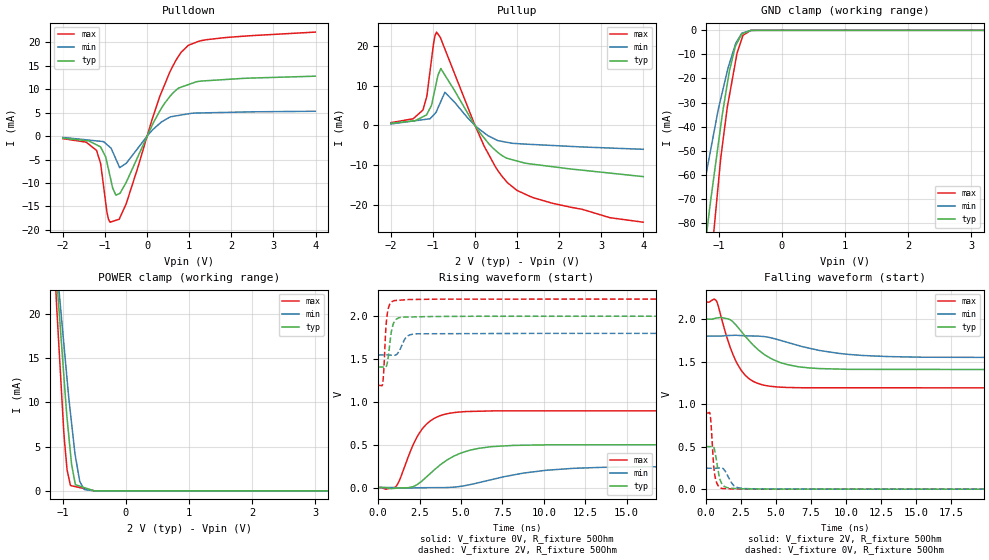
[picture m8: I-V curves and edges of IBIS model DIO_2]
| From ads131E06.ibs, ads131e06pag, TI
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|   DIO 2.0V Model
[Model]   DIO_2
Model_type   I/O
|for ADS1299 products
|Signals   SCLK, DAISY_IN
Vinl = 0.4
Vinh = 1.6
Vmeas = 1
Vref = 1
Cref = 2pF
Rref = 50
|   typ   min   max
|   (nom PVT)   (Fast PVT)   (slow PVT)
|C_comp from LC tank measurement(L=1nH)
|   (HIGH Z)
|C_comp   2.655E-12   2.033E-12   3.282E-12
|   (ON state)
C_comp   2.643E-12   2.033E-12   3.282E-12
|   (OFF state)
|C_comp   2.755E-12   2.168E-12   3.374E-12
| Where   nom PVT is  Nominal Process, 2V, 27C
|   Fast PVT is Strong Process, 2.2V, -40C
|   Slow PVT is Weak Process, 1.8V, 85C
[Voltage Range]   2   1.8   2.2
[Temperature Range]   27   85   -40
[Pullup Reference]   2   1.8   2.2
[Pulldown Reference]   0   0   0
[Power Clamp Reference]   2   1.8   2.2
[GND Clamp Reference]   0   0   0
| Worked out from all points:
|   slope of the pulldown table from 0 to 0.3 V, typ, clamps not added: 56.3 ohm
|   slope of the pullup table from 0 to 0.3 V, typ, clamps not added: 70.4 ohm
|   GND clamp passes 1 mA (typ) near -0.58 V on its own axis
|   POWER clamp passes 1 mA (typ) near -0.81 V on its own axis
|   falling waveform, V_fixture 2V, R_fixture 50Ohm: 20-80 % time 2.39ns typ, 4.11ns min, 1.41ns max; typ from 2 V to 1.41 V
|   rising waveform, V_fixture 0V, R_fixture 50Ohm: 20-80 % time 2.19ns typ, 4.04ns min, 1.33ns max; typ from 0 V to 0.501 V
|   rising waveform, V_fixture 2V, R_fixture 50Ohm: 20-80 % time 260ps typ, 390ps min, 186ps max; typ from 1.41 V to 2 V
|   falling waveform, V_fixture 0V, R_fixture 50Ohm: 20-80 % time 347ps typ, 530ps min, 235ps max; typ from 0.501 V to 0 V
[Pulldown]
|   Voltage   I(typ)   I(min)   I(max)
-2V       -446.8uA   -277.7uA   -546.8uA
-1.45V    -956.7uA   -786.1uA   -1.281mA
-1.202V   -1.858mA   -1.015mA   -3.045mA
-1.101V   -2.393mA   -1.109mA   -6.024mA
-920.3mV  -6.956mA   -2.063mA   -17.66mA
-817.4mV  -11.1mA    -3.341mA   -18.19mA
-664mV    -12.29mA   -6.482mA   -17.75mA
-496.8mV  -9.874mA   -5.806mA   -14.44mA
301.3mV   5.35mA     2.714mA    8.483mA
684.3mV   9.787mA    4.318mA    16.19mA
979.1mV   10.99mA    4.761mA    19.38mA
3.994V    12.79mA    5.303mA    22.2mA
[GND Clamp]
|   Voltage   I(typ)   I(min)   I(max)
-2V       -269mA     -184.2mA   -378.3mA
-1.355V   -119.3mA   -81.26mA   -169.4mA
-1.284V   -104.1mA   -71.39mA   -146.5mA
-1.131V   -71.25mA   -50.04mA   -99.31mA
-1.099V   -65.05mA   -45.58mA   -89.46mA
-1.009V   -47.58mA   -33.04mA   -64.31mA
-946.2mV  -35.5mA    -26.01mA   -48.62mA
-832mV    -17.03mA   -13.86mA   -27.24mA
-712mV    -5.404mA   -4.544mA   -9.78mA
-635mV    -1.555mA   -1.176mA   -3.554mA
-449.5mV  -18.29uA   -16.69uA   -19.05uA
3.994V    0A         0A         0A
[Pullup]
|   Voltage   I(typ)   I(min)   I(max)
-2V       546.5uA    370.9uA    725.3uA
-1.238V   2.207mA    1.461mA    3.888mA
-1.146V   2.755mA    1.593mA    7.345mA
-1.034V   5.103mA    2.08mA     16.64mA
-982.9mV  7.593mA    2.654mA    20.83mA
-913.5mV  11.03mA    3.622mA    23.6mA
-812.5mV  14.38mA    6.062mA    21.93mA
-716.1mV  12.74mA    8.388mA    19.32mA
210.3mV   -3.086mA   -1.805mA   -5.071mA
768.5mV   -8.32mA    -4.277mA   -14.44mA
1.417V    -9.85mA    -4.829mA   -18.36mA
3.994V    -12.92mA   -6.02mA    -24.44mA
[POWER Clamp]
|   Voltage   I(typ)   I(min)   I(max)
-2V       129.9mA    109.1mA    159.1mA
-1.265V   42.77mA    39.99mA    44.99mA
-1.099V   24.37mA    25.59mA    20.8mA
-1.077V   21.95mA    23.81mA    18.06mA
-978.4mV  12.37mA    16.1mA     5.936mA
-933.4mV  8.162mA    12.58mA    2.352mA
-879.9mV  4.267mA    8.781mA    608.5uA
-862.6mV  3.01mA     7.665mA    581.1uA
-802.3mV  700.9uA    3.939mA    485.3uA
-735.2mV  546.5uA    1.154mA    378.6uA
-660.5mV  374.8uA    150.3uA    260uA
3.994V    0A         0A         0A
[Ramp]
R_load = 50
|   typ   min   max
dV/dt_r   0.300352/2.17829e-009  0.147656/3.99197e-009  0.537699/1.32728e-009
dV/dt_f   0.356044/2.37937e-009  0.151292/4.09875e-009  0.605232/1.41384e-009
[Falling Waveform]
V_fixture = 2V
V_fixture_min = 1.8V
V_fixture_max = 2.2V
R_fixture = 50Ohm
C_fixture = 0F
|   Time   V(typ)   V(min)   V(max)
0s        2V         1.8V       2.2V
749.6ps   2.013V     1.8V       2.209V
1.715ns   1.993V     1.808V     1.671V
2.488ns   1.86V      1.806V     1.403V
3.156ns   1.732V     1.802V     1.289V
4.022ns   1.601V     1.796V     1.227V
5.876ns   1.462V     1.724V     1.196V
8.072ns   1.418V     1.632V     1.193V
13.08ns   1.409V     1.559V     1.192V
25ns      1.407V     1.548V     1.191V
[Rising Waveform]
V_fixture = 0V
V_fixture_min = 0V
V_fixture_max = 0V
R_fixture = 50Ohm
C_fixture = 0F
|   Time   V(typ)   V(min)   V(max)
0s        184.8nV    7.826uV    109.4nV
1.066ns   -7.55mV    -987.3uV   11.36mV
2.103ns   9.758mV    -4.291mV   495.5mV
2.606ns   70.92mV    -2.049mV   669.5mV
3.326ns   195.8mV    -1.253mV   800.9mV
4.291ns   336.3mV    1.801mV    866.6mV
5.482ns   433mV      31.63mV    888mV
6.745ns   475.1mV    87.79mV    893.8mV
11.72ns   498.8mV    223.4mV    895.2mV
25ns      500.6mV    246.1mV    896.2mV
[Rising Waveform]
V_fixture = 2V
V_fixture_min = 1.8V
V_fixture_max = 2.2V
R_fixture = 50Ohm
C_fixture = 0F
|   Time   V(typ)   V(min)   V(max)
0s        1.407V     1.548V     1.191V
278.5ps   1.406V     1.548V     1.226V
347.1ps   1.404V     1.548V     1.401V
466.8ps   1.408V     1.548V     1.865V
585.2ps   1.496V     1.548V     2.068V
785ps     1.806V     1.545V     2.162V
992.4ps   1.941V     1.544V     2.183V
1.707ns   1.99V      1.758V     2.193V
2.323ns   1.992V     1.795V     2.196V
25ns      2V         1.8V       2.2V
[Falling Waveform]
|Gnd
V_fixture = 0V
V_fixture_min = 0V
V_fixture_max = 0V
R_fixture = 50Ohm
C_fixture = 0F
|   Time   V(typ)   V(min)   V(max)
0s        500.6mV    246.1mV    896.2mV
293.9ps   500.4mV    246.1mV    873.4mV
362.6ps   502.7mV    246mV      744.6mV
536.9ps   496mV      246mV      287.3mV
659.2ps   416.6mV    246mV      130.6mV
925.9ps   159.4mV    249.2mV    26.41mV
1.119ns   65.38mV    249.3mV    9.224mV
1.981ns   8.501mV    42.39mV    2.845mV
2.757ns   3.635mV    7.2mV      1.894mV
25ns      274.3nV    8.023uV    171.3nV
